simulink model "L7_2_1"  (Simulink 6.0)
settings: Solver=ode5  StartTime=0.0  StopTime=10.0  RelTol=1e-3
libraries: simulink x1

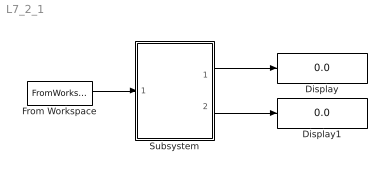
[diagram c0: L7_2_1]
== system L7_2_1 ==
  Display : Display
  Display1 : Display
  From Workspace : FromWorkspace  VariableName=x  SampleTime=0
  Subsystem : Subsystem
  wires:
  From Workspace/1 -> Subsystem/1(In1)
  Subsystem/1(Out1) -> Display/1
  Subsystem/2(Out2) -> Display1/1

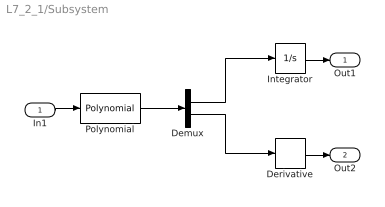
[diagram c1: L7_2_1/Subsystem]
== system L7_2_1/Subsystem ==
  In1 : Inport  Port=1  LatchInput=off
  Demux : Demux  Outputs=2
  Derivative : Derivative
  Integrator : Integrator
  Polynomial : simulink/Math Operations/Polynomial  coefs=[1 2 4 1]
  Out1 : Outport
  Out2 : Outport  Port=2
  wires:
  Polynomial/1 -> Demux/1
  Demux/1 -> Integrator/1
  Demux/2 -> Derivative/1
  Integrator/1 -> Out1/1
  In1/1 -> Polynomial/1
  Derivative/1 -> Out2/1
